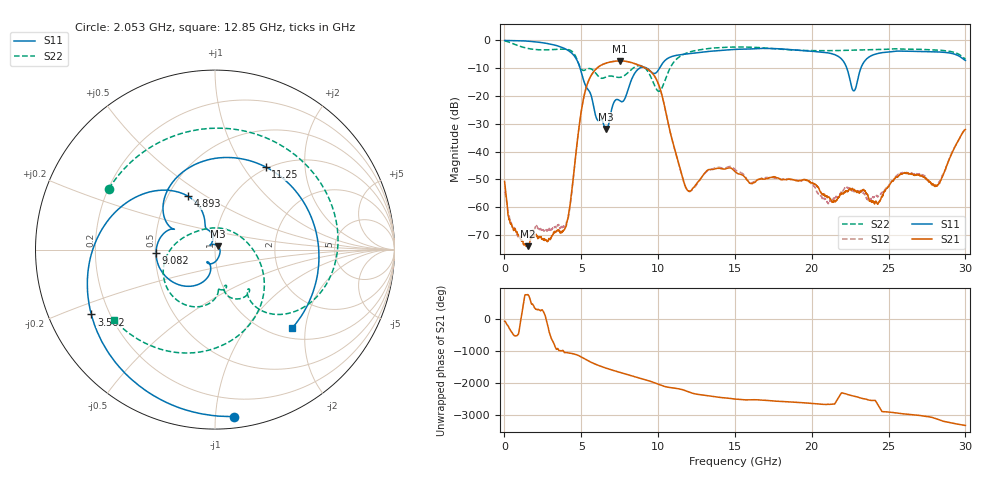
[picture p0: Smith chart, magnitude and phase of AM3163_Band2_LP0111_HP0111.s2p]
!Agilent Technologies,E8364B,MY43040894,A.07.50.67
!Agilent E8364B: A.07.50.67
!Date: Thursday, August 20, 2020 11:12:56
!Correction: S11(Full 2 Port(1,2))
!S21(Full 2 Port(1,2))
!S12(Full 2 Port(1,2))
!S22(Full 2 Port(1,2))
!S2P File: Measurements: S11, S21, S12, S22:
# Hz S  dB  R 50
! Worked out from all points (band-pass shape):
!   3201 points, 10 MHz to 30 GHz, reference 50 ohm
!   highest |S21| = -7.39 dB at 7.517 GHz (marker M1); lowest = -74.1 dB at 1.51 GHz (marker M2)
!   |S21| within 3 dB of the highest: 5.945 GHz to 9.312 GHz (3.367 GHz wide, 44.1 % of centre)
!   lowest |S11| = -31.9 dB at 6.617 GHz (marker M3), VSWR 1.05, Z = 51.8 + j1.89 ohm
!   |S11| at or under -10 dB: 4.923 GHz to 8.8 GHz (3.877 GHz wide, 56.5 % of centre); 9.256 GHz to 10.09 GHz (835.9 MHz wide, 8.64 % of centre); 22.28 GHz to 23.2 GHz (913.9 MHz wide, 4.02 % of centre)
!   |S22| runs from -18.3 to -0.2 dB; largest |S21 - S12| = 0.0038
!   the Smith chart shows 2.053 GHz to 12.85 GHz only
!   S11 on the Smith chart (normalised r, x): 2.053 GHz: 0.07, -1.12; 3.562 GHz: 0.13, -0.24; 4.893 GHz: 0.63, +0.42; 9.082 GHz: 0.51, -0.02; 11.25 GHz: 0.97, +1.27; 12.85 GHz: 1.20, -1.69
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1e7  -0.04 -2.7  -50.78 -62.0  -54.42 -81.4  -0.22 -9.4
6.660312e8  -0.09 -26.6  -67.77 -161.4  -67.68 -102.2  -1.45 -85.3
1.5095e9  -0.30 -60.8  -74.06 48.0  -69.81 160.3  -2.89 -167.1
2.053069e9  -0.57 -83.4  -69.72 -48.5  -67.15 75.9  -3.33 150.1
3.561941e9  -2.18 -152.3  -68.33 98.5  -67.10 -53.5  -3.19 44.5
4.161741e9  -3.69 173.1  -62.86 24.3  -63.68 14.8  -3.34 -1.6
4.892747e9  -9.48 117.1  -29.59 -74.0  -29.62 -74.2  -9.26 -55.4
5.014581e9  -11.73 110.2  -24.98 -105.0  -25.01 -105.3  -10.41 -53.3
6.617172e9  -31.90 45.7  -8.19 -90.7  -8.21 -90.8  -13.17 -73.2
7.516872e9  -21.78 -123.2  -7.39 137.1  -7.42 137.0  -13.33 -85.7
8.369712e9  -12.92 -118.3  -8.18 20.3  -8.20 20.3  -10.01 -100.1
9.081975e9  -9.66 -176.9  -9.72 -77.0  -9.74 -77.0  -9.65 -149.3
1.000979e10  -10.74 152.6  -15.58 129.0  -15.53 128.8  -18.28 99.9
1.124688e10  -5.35 58.4  -42.40 -7.9  -42.69 -8.6  -6.51 -68.5
1.284947e10  -4.24 -45.6  -49.23 154.3  -49.12 159.9  -3.28 -145.1
1.5005e10  -3.27 -141.8  -47.20 24.2  -46.40 24.8  -2.40 137.9
1.773222e10  -3.01 94.8  -49.49 -43.0  -49.76 -42.8  -3.10 33.2
2.000958e10  -3.95 -25.8  -51.34 -113.2  -51.93 -122.6  -3.70 -48.8
2.27368e10  -18.17 -109.1  -53.96 115.3  -54.41 121.6  -3.54 -126.3
2.500479e10  -4.17 -150.6  -52.66 -21.9  -52.23 -24.2  -3.22 178.0
2.816311e10  -4.16 110.6  -52.37 120.2  -52.28 122.5  -3.47 94.0
3e10  -7.21 44.2  -32.05 -79.8  -31.89 -77.0  -6.70 37.5
